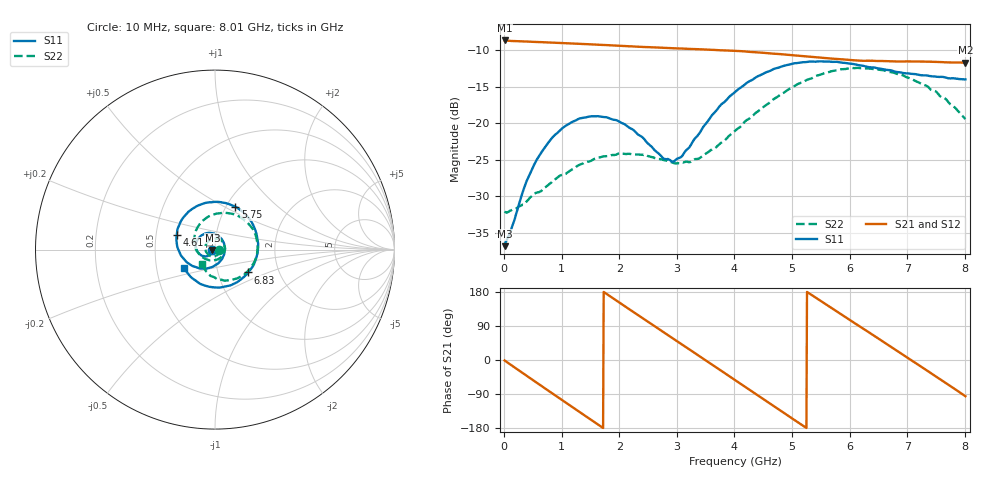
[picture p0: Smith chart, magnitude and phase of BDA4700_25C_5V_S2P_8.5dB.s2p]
!Agilent Technologies,E5071B,MY42404982,A.09.10
!Date: Mon Oct 20 13:30:16 2025
!Data & Calibration Information:
!Freq	S11:SOLT2(ON)	S21:SOLT2(ON)	S12:SOLT2(ON)	S22:SOLT2(ON)
# Hz S RI R 50
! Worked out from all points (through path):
!   801 points, 10 MHz to 8.01 GHz, reference 50 ohm
!   highest |S21| = -8.62 dB at 10 MHz (marker M1); lowest = -11.7 dB at 8.01 GHz (marker M2)
!   group delay of S21, straight-line fit = 282 ps
!   lowest |S11| = -36.9 dB at 10 MHz (marker M3), VSWR 1.03, Z = 48.6 - j0.157 ohm
!   |S11| at or under -10 dB: start of sweep to end of sweep
!   |S22| runs from -32.3 to -12.4 dB; largest |S21 - S12| = 0.0026
!   S11 on the Smith chart (normalised r, x): 10 MHz: 0.97, -0.00; 4.61 GHz: 0.64, +0.11; 5.75 GHz: 1.10, +0.57; 6.83 GHz: 1.40, -0.37; 8.01 GHz: 0.69, -0.15
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1e7  -0.0142 -0.00161  0.3705 -0.00812  0.3705 -0.00855  0.0248 -0.00135
4e8  -0.028 -0.0295  0.269 -0.2454  0.2688 -0.2459  0.0187 -0.0226
7.2e8  -0.0583 -0.0374  0.0882 -0.3487  0.0882 -0.349  -0.00116 -0.0364
1.02e9  -0.0906 -0.0212  -0.1036 -0.3402  -0.1041 -0.3403  -0.029 -0.0335
1.35e9  -0.107 0.0196  -0.2734 -0.2201  -0.2735 -0.2202  -0.0523 -0.00501
1.64e9  -0.0938 0.061  -0.3423 -0.0535  -0.3425 -0.0535  -0.05 0.0296
1.93e9  -0.0568 0.0889  -0.3192 0.1221  -0.3193 0.1224  -0.0235 0.0559
2.32e9  0.00616 0.0838  -0.1638 0.2932  -0.1636 0.2935  0.0258 0.0554
2.68e9  0.0485 0.0389  0.0429 0.3284  0.0428 0.3283  0.0541 0.0176
2.96e9  0.0533 -0.014  0.1919 0.2652  0.192 0.2648  0.0498 -0.0185
3.37e9  0.00865 -0.0827  0.315 0.0694  0.3155 0.0691  0.00915 -0.0562
3.68e9  -0.0607 -0.1054  0.3009 -0.1045  0.3009 -0.1054  -0.0365 -0.0577
4.01e9  -0.1429 -0.0803  0.1893 -0.2509  0.1895 -0.2508  -0.0828 -0.0321
4.61e9  -0.2136 0.0818  -0.1252 -0.2754  -0.1248 -0.2758  -0.1127 0.081
5e9  -0.1553 0.2036  -0.2637 -0.1283  -0.2645 -0.1287  -0.0637 0.1645
5.35e9  -0.0403 0.2623  -0.2817 0.0469  -0.282 0.0462  0.0282 0.2026
5.75e9  0.1136 0.239  -0.1804 0.2103  -0.1801 0.2104  0.1484 0.1762
6.2e9  0.2257 0.1054  0.0174 0.2685  0.0195 0.269  0.2322 0.0575
6.68e9  0.2184 -0.0782  0.2081 0.1667  0.2087 0.1665  0.2078 -0.088
6.83e9  0.1856 -0.127  0.243 0.1073  0.2437 0.1065  0.1798 -0.1226
7.34e9  0.0209 -0.212  0.2351 -0.1222  0.2353 -0.1225  0.0512 -0.1728
8.01e9  -0.1723 -0.1021  -0.0258 -0.2595  -0.0255 -0.2598  -0.0722 -0.0788
